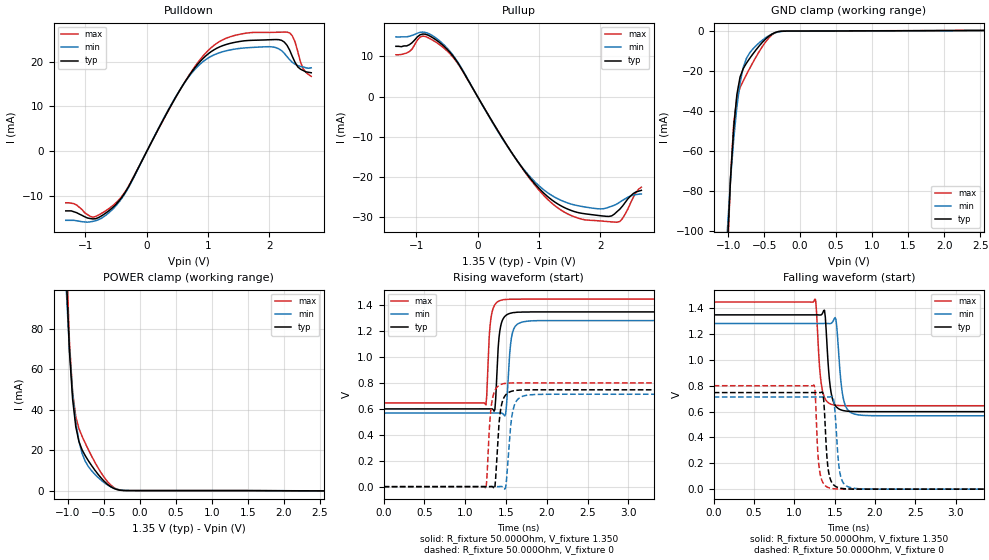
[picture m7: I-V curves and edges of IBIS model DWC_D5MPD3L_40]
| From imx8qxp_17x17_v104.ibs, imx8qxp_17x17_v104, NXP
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[Model] DWC_D5MPD3L_40
Model_type   I/O
Polarity   Non-Inverting
Enable   Active-High
C_comp   1.451pF   1.359pF   1.565pF
C_comp_pullup   315.783fF   294.189fF   344.067fF
C_comp_pulldown 1.109pF   1.032pF   1.207pF
Vinh = 800.000mV
Vinl = 550.000mV
Vmeas = 675.000mV
Vref = 675.000mV
Rref = 50Ohms
Cref = 0pF
[Model Spec]
Vinh   800.000mV   767.000mV   850.000mV
Vinl   550.000mV   517.000mV   600.000mV
Vmeas   675.000mV   642.000mV   725.000mV
Vref   675.000mV   642.000mV   725.000mV
D_overshoot_ampl_h 0.4 NA   NA
D_overshoot_ampl_l 0.4 NA   NA
D_overshoot_area_l 100.000p NA   NA
D_overshoot_area_h 100.000p NA   NA
[Receiver Thresholds]
Vcross_low = 525.000mV
Vcross_high = 825.000mV
Vdiff_ac = 250.000mV
Vdiff_dc = 180.000mV
Tdiffslew_ac = 10.000ns
[Temperature Range]   25.000   125.000   -40.000
[Voltage Range]   1.350V   1.283V   1.450V
[GND Clamp Reference]   0.00V   0.00V   0.00V
[Pulldown Reference]   0.00V   0.00V   0.00V
[POWER Clamp Reference]   1.350V   1.283V   1.450V
[Pullup Reference]   1.350V   1.283V   1.450V
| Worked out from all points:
|   slope of the pulldown table from 0 to 0.203 V, typ, clamps not added: 38 ohm
|   slope of the pullup table from 0 to 0.203 V, typ, clamps not added: 38.5 ohm
|   GND clamp passes 1 mA (typ) near -0.36 V on its own axis
|   POWER clamp passes 1 mA (typ) near -0.36 V on its own axis
|   rising waveform, R_fixture 50.000Ohm, V_fixture 1.350: 20-80 % time 44.3ps typ, 49.1ps min, 42.1ps max; typ from 0.599 V to 1.35 V
|   rising waveform, R_fixture 50.000Ohm, V_fixture 0: 20-80 % time 53.8ps typ, 62.2ps min, 50.1ps max; typ from 0 V to 0.746 V
|   falling waveform, R_fixture 50.000Ohm, V_fixture 1.350: 20-80 % time 57.8ps typ, 64.5ps min, 54.5ps max; typ from 1.35 V to 0.599 V
|   falling waveform, R_fixture 50.000Ohm, V_fixture 0: 20-80 % time 47.2ps typ, 53.7ps min, 43.3ps max; typ from 0.746 V to 0 V
[GND Clamp]
-1.318V   -611.9mA   -435.6mA   -789.4mA
-1.011V   -107.3mA   -99.44mA   -114.7mA
-966.7mV  -73.21mA   -74.14mA   -72.86mA
-922.7mV  -48.19mA   -53.84mA   -45.97mA
-878.8mV  -31.65mA   -37.83mA   -33.26mA
-834.8mV  -22.94mA   -25.98mA   -28.23mA
-790.9mV  -18.78mA   -18.21mA   -24.87mA
-747mV    -16.07mA   -13.69mA   -21.78mA
-483.3mV  -4.069mA   -3.422mA   -5.579mA
-351.5mV  -769.8uA   -913.6uA   -898.3uA
-263.6mV  -80.12uA   -193.4uA   -52.02uA
2.68V     309.8uA    252.8uA    386uA
[Power Clamp]
-1.33V    624.3mA    459.2mA    781.3mA
-1.023V   106.8mA    99.48mA    118.2mA
-978.8mV  68.81mA    69.68mA    73.53mA
-934.8mV  45.17mA    48.25mA    48.62mA
-890.9mV  31.58mA    33.85mA    36.56mA
-847mV    24.24mA    24.41mA    30.7mA
-803mV    20.11mA    18.35mA    26.81mA
-715.2mV  14.71mA    11.84mA    20.17mA
-451.5mV  3.129mA    2.823mA    4.473mA
-363.6mV  1.086mA    1.21mA     1.534mA
-231.8mV  46.56uA    141.6uA    53.57uA
2.668V    -152.4uA   -131.4uA   -175.4uA
[Pulldown]
-1.318V   -13.2mA    -15.3mA    -11.4mA
-878.8mV  -14.99mA   -15.54mA   -14.61mA
-483.3mV  -11.5mA    -11.78mA   -11.17mA
-307.6mV  -8.113mA   -8.287mA   -7.978mA
615.2mV   15.29mA    15.24mA    15.33mA
922.7mV   20.75mA    20.02mA    21.3mA
1.23V     23.48mA    22.14mA    24.77mA
2.065V    24.86mA    23.21mA    26.48mA
2.329V    22.52mA    20.4mA     26.35mA
2.417V    19.8mA     19.4mA     24.33mA
2.549V    18mA       18.8mA     18.4mA
2.68V     17.5mA     18.6mA     16.7mA
[Pullup]
-1.33V    12.5mA     14.85mA    10.4mA
-1.111V   12.9mA     15.01mA    11.19mA
-890.9mV  15.56mA    16.04mA    15.04mA
-495.5mV  11.76mA    12.05mA    11.35mA
-275.8mV  7.283mA    7.45mA     7.139mA
690.9mV   -16.93mA   -16.85mA   -17mA
1.086V    -24.09mA   -23.26mA   -24.67mA
1.438V    -27.75mA   -26.26mA   -28.91mA
2.141V    -29.77mA   -27.47mA   -31.08mA
2.317V    -27.98mA   -26.22mA   -31.04mA
2.536V    -24.1mA    -24.5mA    -25.06mA
2.668V    -23.3mA    -24.2mA    -22.51mA
[Ramp]
R_load=50.000Ohm
dV/dt_r   448.110mV/50.000ps  427.618mV/56.500ps  479.910mV/46.500ps
dV/dt_f   448.110mV/53.000ps  427.618mV/59.500ps  479.910mV/50.000ps
[Rising waveform]
R_fixture=50.000Ohm
V_fixture=1.350
V_fixture_min=1.283
V_fixture_max=1.450
0s        599.3mV    567.4mV    645.4mV
1.253ns   599.3mV    567.3mV    630.7mV
1.323ns   600.4mV    567.4mV    1.329V
1.363ns   595.1mV    567.2mV    1.403V
1.413ns   1.146V     568.2mV    1.431V
1.474ns   1.304V     552.6mV    1.442V
1.504ns   1.323V     615.6mV    1.443V
1.574ns   1.34V      1.174V     1.445V
1.764ns   1.346V     1.276V     1.446V
10ns      1.347V     1.28V      1.446V
[Rising waveform]
R_fixture=50.000Ohm
V_fixture=0
0s        384.3nV    8.074uV    52.65nV
1.253ns   7.701uV    4.453uV    -15.16mV
1.303ns   257uV      15.14uV    520.9mV
1.333ns   357.2uV    14.82uV    677.8mV
1.363ns   -4.772mV   -72.94uV   740.8mV
1.434ns   596mV      1.525mV    787.2mV
1.494ns   706.2mV    -8.025mV   796.4mV
1.584ns   738.3mV    587mV      799.7mV
1.774ns   746.4mV    706.4mV    800.2mV
10ns      746.3mV    712.3mV    799.6mV
[Falling waveform]
R_fixture=50.000Ohm
V_fixture=1.350
V_fixture_min=1.283
V_fixture_max=1.450
0s        1.347V     1.28V      1.446V
1.253ns   1.347V     1.28V      1.469V
1.313ns   1.346V     1.28V      934.3mV
1.343ns   1.353V     1.28V      776mV
1.373ns   1.383V     1.281V     709mV
1.434ns   847.4mV    1.279V     662.1mV
1.504ns   649.3mV    1.326V     648.8mV
1.614ns   606.2mV    680.9mV    645mV
1.794ns   599.2mV    573.9mV    644.5mV
10ns      599.2mV    567.3mV    645.2mV
[Falling waveform]
R_fixture=50.000Ohm
V_fixture=0
0s        746.2mV    712.2mV    799.4mV
1.243ns   746.2mV    712.2mV    804.6mV
1.253ns   746.2mV    712.2mV    786.1mV
1.313ns   745.9mV    712.2mV    139.5mV
1.353ns   743.1mV    712.2mV    50.82mV
1.413ns   182.9mV    711.8mV    14.03mV
1.474ns   41.66mV    716.8mV    4.045mV
1.574ns   7.285mV    98.05mV    558uV
1.744ns   473.2uV    6.331mV    44.78uV
10ns      425.6nV    8.256uV    263.1nV
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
